DATA_BLOCK DB 18
AUTHOR : Esposito
FAMILY : EGAL_srl
NAME : STATUS_L
VERSION : 0.1


  STRUCT
   Car_st_co_1 : BOOL ;	//Pomp wagon in march.
   Car_st_co_2 : BOOL ;	//Presence coil in the store.
   Car_st_co_3 : BOOL ;	//Presence coil on the wagon.
   Car_st_co_4 : BOOL ;	//Wagon in the store.
   Car_st_co_5 : BOOL ;	//Wagon out of the store.
   Car_st_co_6 : BOOL ;	//Wagon zone reel.
   Car_st_co_7 : BOOL ;	//Cylinder tall wagon.
   Car_st_co_8 : BOOL ;	//Cylinder low wagon.
   Car_st_co_9 : BOOL ;	//Not alarms wagon.
   Car_st_co_10 : BOOL ;	//Spare for status wagon, store, and coil.
   Car_st_co_11 : BOOL ;	//Spare for status wagon, store, and coil.
   Car_st_co_12 : BOOL ;	//Spare for status wagon, store, and coil.
   Car_st_co_13 : BOOL ;	//Spare for status wagon, store, and coil.
   Car_st_co_14 : BOOL ;	//Spare for status wagon, store, and coil.
   Car_st_co_15 : BOOL ;	//Spare for status wagon, store, and coil.
   Car_st_co_16 : BOOL ;	//Spare for status wagon, store, and coil.
   Reel_1 : BOOL ;	//Mandrel front out.
   Reel_2 : BOOL ;	//Mandrel front inside.
   Reel_3 : BOOL ;	//Rolls tall pressure.
   Reel_4 : BOOL ;	//Mandrel front pressure ok.
   Reel_5 : BOOL ;	//carrying out coil from above.
   Reel_6 : BOOL ;	//carrying out coil from under.
   Reel_7 : BOOL ;	//Mandrel rear out.
   Reel_8 : BOOL ;	//Mandrel rear inside.
   Reel_9 : BOOL ;	//Inserted draught.
   Reel_10 : BOOL ;	//Mandrel rear pressure ok.
   Reel_11 : BOOL ;	//Not alarms reel.
   Reel_12 : BOOL ;	//Spare for status reel.
   Reel_13 : BOOL ;	//Spare for status reel.
   Reel_14 : BOOL ;	//Spare for status reel.
   Reel_15 : BOOL ;	//Spare for status reel.
   Reel_16 : BOOL ;	//Spare for status reel.
   Straightener_1 : BOOL ;	//Compenetration entry side all open.
   Straightener_2 : BOOL ;	//Compenetration entry side all closed.
   Straightener_3 : BOOL ;	//Pinch roll open entry.
   Straightener_4 : BOOL ;	//Blankcart present entry.
   Straightener_5 : BOOL ;	//Pomp lubrication oil march
   Straightener_6 : BOOL ;	//Automatic inserted.
   Straightener_7 : BOOL ;	//Straightener inserted.
   Straightener_8 : BOOL ;	//Not alarms straightener.
   Straightener_9 : BOOL ;	//Compenetration exit side all open.
   Straightener_10 : BOOL ;	//Compenetration exit side all closed.
   Straightener_11 : BOOL ;	//Pinch roll exit open.
   Straightener_12 : BOOL ;	//Blankcart present exit.
   Straightener_13 : BOOL ;	//Spare for status straightener.
   Straightener_14 : BOOL ;	//Spare for status straightener.
   Straightener_15 : BOOL ;	//Spare for status straightener.
   Straightener_16 : BOOL ;	//Spare for status straightener.
   Ansa_1 : BOOL ;	//Short Handle (alarm)
   Ansa_2 : BOOL ;	//Short Handle (accelerate)
   Ansa_3 : BOOL ;	//Low Handle (slow down)
   Ansa_4 : BOOL ;	//Low Handle (halt straightener)
   Ansa_5 : BOOL ;	//Guides open blankcart
   Ansa_6 : BOOL ;	//Spare for status handle.
   Ansa_7 : BOOL ;	//Spare for status handle.
   Ansa_8 : BOOL ;	//Spare for status handle.
   Ansa_9 : BOOL ;	//Spare for status handle.
   Ansa_10 : BOOL ;	//Spare for status handle.
   Ansa_11 : BOOL ;	//Spare for status handle.
   Ansa_12 : BOOL ;	//Spare for status handle.
   Ansa_13 : BOOL ;	//Spare for status handle.
   Ansa_14 : BOOL ;	//Spare for status handle.
   Ansa_15 : BOOL ;	//Spare for status handle.
   Ansa_16 : BOOL ;	//Spare for status handle.
   Feeder_1 : BOOL ;	//Rolls of don't return open.
   Feeder_2 : BOOL ;	//Rolls of open measure.
   Feeder_3 : BOOL ;	//Rolls open feeding.
   Feeder_4 : BOOL ;	//Brake roll decontrolled feeding.
   Feeder_5 : BOOL ;	//Pass line all up.
   Feeder_6 : BOOL ;	//Pass line all down.
   Feeder_7 : BOOL ;	//Jammed feeder.
   Feeder_8 : BOOL ;	//Presence blankcart.
   Feeder_9 : BOOL ;	//Automatic inserted.
   Feeder_10 : BOOL ;	//Inserted Feeder.
   Feeder_11 : BOOL ;	//Not alarms feeder.
   Feeder_12 : BOOL ;	//Spare for status feeder.
   Feeder_13 : BOOL ;	//Spare for status feeder.
   Feeder_14 : BOOL ;	//Spare for status feeder.
   Feeder_15 : BOOL ;	//Spare for status feeder.
   Feeder_16 : BOOL ;	//Spare for status feeder.
  END_STRUCT ;
BEGIN
   Car_st_co_1 := FALSE;
   Car_st_co_2 := FALSE;
   Car_st_co_3 := FALSE;
   Car_st_co_4 := FALSE;
   Car_st_co_5 := FALSE;
   Car_st_co_6 := FALSE;
   Car_st_co_7 := FALSE;
   Car_st_co_8 := FALSE;
   Car_st_co_9 := FALSE;
   Car_st_co_10 := FALSE;
   Car_st_co_11 := FALSE;
   Car_st_co_12 := FALSE;
   Car_st_co_13 := FALSE;
   Car_st_co_14 := FALSE;
   Car_st_co_15 := FALSE;
   Car_st_co_16 := FALSE;
   Reel_1 := FALSE;
   Reel_2 := FALSE;
   Reel_3 := FALSE;
   Reel_4 := FALSE;
   Reel_5 := FALSE;
   Reel_6 := FALSE;
   Reel_7 := FALSE;
   Reel_8 := FALSE;
   Reel_9 := FALSE;
   Reel_10 := FALSE;
   Reel_11 := FALSE;
   Reel_12 := FALSE;
   Reel_13 := FALSE;
   Reel_14 := FALSE;
   Reel_15 := FALSE;
   Reel_16 := FALSE;
   Straightener_1 := FALSE;
   Straightener_2 := FALSE;
   Straightener_3 := FALSE;
   Straightener_4 := FALSE;
   Straightener_5 := FALSE;
   Straightener_6 := FALSE;
   Straightener_7 := FALSE;
   Straightener_8 := FALSE;
   Straightener_9 := FALSE;
   Straightener_10 := FALSE;
   Straightener_11 := FALSE;
   Straightener_12 := FALSE;
   Straightener_13 := FALSE;
   Straightener_14 := FALSE;
   Straightener_15 := FALSE;
   Straightener_16 := FALSE;
   Ansa_1 := FALSE;
   Ansa_2 := FALSE;
   Ansa_3 := FALSE;
   Ansa_4 := FALSE;
   Ansa_5 := FALSE;
   Ansa_6 := FALSE;
   Ansa_7 := FALSE;
   Ansa_8 := FALSE;
   Ansa_9 := FALSE;
   Ansa_10 := FALSE;
   Ansa_11 := FALSE;
   Ansa_12 := FALSE;
   Ansa_13 := FALSE;
   Ansa_14 := FALSE;
   Ansa_15 := FALSE;
   Ansa_16 := FALSE;
   Feeder_1 := FALSE;
   Feeder_2 := FALSE;
   Feeder_3 := FALSE;
   Feeder_4 := FALSE;
   Feeder_5 := FALSE;
   Feeder_6 := FALSE;
   Feeder_7 := FALSE;
   Feeder_8 := FALSE;
   Feeder_9 := FALSE;
   Feeder_10 := FALSE;
   Feeder_11 := FALSE;
   Feeder_12 := FALSE;
   Feeder_13 := FALSE;
   Feeder_14 := FALSE;
   Feeder_15 := FALSE;
   Feeder_16 := FALSE;
END_DATA_BLOCK

